FUNCTION_BLOCK JsonObjV5
VAR_INPUT
END_VAR
VAR_OUTPUT
END_VAR
VAR
	// json功能块
	fbJsonRWDT : FB_JsonReadWriteDataType;
	fbJsonW : FB_JsonSaxWriter;
	fbJsonDP : FB_JsonDomParser;
	// 保存出的json字符串
	jsonStr : STRING(255);
	// json键值对地址
	ArrAdr : INT;
	// 键数组
	keyArr : ARRAY[0..999] OF STRING;
	// 值数组
	dataArr : ARRAY[0..999] OF STRING(255);
	// 值数据类型-未启用
	typeArr : ARRAY[0..999] OF STRING;
END_VAR

(*
* 功能 1 输入键（字符串）-值（任意数据类型）自动载入json
* 功能 2 输入键（字符串）自动返回值（任意数据类型，包括自定义数据类型以及JSON）
* 功能 3 JSON数据重置
* 功能 4 输出JSON字符串
* 功能 5 输入JSON字符串，转化为Json对象
* 功能 6 输入特定结构体对象，直接转化为Json字符串并返回
* 功能 7 输入JSON字符串，转化为结构体
*)

METHOD AddKeyValue : BOOL
VAR_INPUT
	key : STRING;// JSON键
 	nData : UDINT;// 值变量长度
 	pData : PVOID;// 值变量起始地址
END_VAR
VAR
	typestr : STRING;// 值变量数据类型
	tempstr : STRING;// 临时字符串变量
	keystr : STRING;// 键临时变量
END_VAR
(*
* 功能 1 输入键（字符串）-值（任意数据类型）自动载入json
*)
// 获得值变量的数据类型
typestr := fbJsonRWDT.GetDatatypeNameByAddress(nData := nData, pData := pData);
// 重置Json缓存
fbJsonW.ResetDocument();
// 添加数据到Json缓存
fbJsonRWDT.AddJsonValueFromSymbol(fbJsonW, typestr, nData, pData);
// 将当前缓存转为字符串
tempstr := fbJsonW.GetDocument();
// 将键转换为键格式
keystr := concat('"', concat(key, '"'));
// 写入数组缓存
keyArr[ArrAdr] := keystr;
dataArr[ArrAdr] := tempstr;
typeArr[ArrAdr] := typestr;
// 地址+1
ArrAdr := ArrAdr + 1;
END_METHOD

METHOD GetJsonStr : string(1000)
VAR_INPUT
END_VAR
VAR
	i: INT;
END_VAR
(*
* 功能 4 输出JSON字符串
*)
// 起始大括号
GetJsonStr := Tc2_Standard.CONCAT(GetJsonStr, '{');
// 遍历数据数组
FOR i := 0 TO ArrAdr - 1 BY 1 DO
	// 第二个元素开始要加上逗号分隔
	IF i > 0 THEN
		GetJsonStr := Tc2_Standard.CONCAT(GetJsonStr, ',');
	END_IF
	// 拼接键
	GetJsonStr := Tc2_Standard.CONCAT(GetJsonStr, KeyArr[i]);
	// 冒号分隔
	GetJsonStr := Tc2_Standard.CONCAT(GetJsonStr, ':');
	// 拼接值
	GetJsonStr := Tc2_Standard.CONCAT(GetJsonStr, dataArr[i]);
END_FOR
// 末尾大括号
GetJsonStr := Tc2_Standard.CONCAT(GetJsonStr, '}');
END_METHOD

METHOD GetKeyValue : BOOL
VAR_INPUT
	key : STRING;// JSON键
 	nData : UDINT;// 值变量返回长度
 	pData : PVOID;// 值变量返回起始地址
END_VAR
VAR
	typestr : STRING;// 值变量数据类型
	i : INT;// 键值
	sJson : string(255);
END_VAR
(*
* 功能 2 输入键（字符串）自动返回值（任意数据类型，包括自定义数据类型以及JSON）
*)
// Json中是否存在数据
IF arradr > 0 THEN
	// 获得值变量的数据类型
	typestr := fbJsonRWDT.GetDatatypeNameByAddress(nData := nData, pData := pData);
	// 遍历查找键值
	FOR i := 0 TO ArrAdr - 1 BY 1 DO
		// 给key拼接上""，判断键是否相等
		IF keyarr[i] = concat('"', concat(key, '"')) THEN
			// 如果相等，则返回值
			fbJsonRWDT.SetSymbolFromJson(sJson:= dataarr[i], sDatatype:= typestr, nData := nData, pData := pData);
			EXIT;
		END_IF
	END_FOR
END_IF
END_METHOD

METHOD JsonStrToObj : bool
VAR_INPUT
	JsonStr: STRING(1000);
	nData: UDINT;
	pData: PVOID;
END_VAR
VAR
	typestr: STRING;
END_VAR
(*
* 功能 7 输入JSON字符串，转化为结构体
*)
// 获得值变量的数据类型
typestr := fbJsonRWDT.GetDatatypeNameByAddress(nData := nData, pData := pData);
// 重置Json缓存
fbJsonW.ResetDocument();
// 将JSON字符串的信息写入特定数据
fbJsonRWDT.SetSymbolFromJson(sJson:= JsonStr, sDatatype:= typestr, nData:= nData, pData:= pData);
END_METHOD

METHOD ObjToJsonStr : STRING(1000)
VAR_INPUT
	nData: UDINT;
	pData: PVOID;
END_VAR
VAR
	typestr: STRING;
END_VAR
(*
* 功能 6 输入特定结构体对象，直接转化为Json字符串并返回
*)
// 获得值变量的数据类型
typestr := fbJsonRWDT.GetDatatypeNameByAddress(nData := nData, pData := pData);
// 重置Json缓存
fbJsonW.ResetDocument();
// 添加数据到Json缓存
fbJsonRWDT.AddJsonValueFromSymbol(fbJsonW, typestr, nData, pData);
// 将当前缓存转为字符串
fbJsonW.CopyDocument(pDoc:= ObjToJsonStr, nDoc:= SIZEOF(ObjToJsonStr));
END_METHOD

METHOD ResetObj : BOOL
VAR_INPUT
END_VAR
(*
* 功能 3 JSON数据重置
*)
// json键值对地址重置为0
ArrAdr := 0;
END_METHOD

END_FUNCTION_BLOCK
